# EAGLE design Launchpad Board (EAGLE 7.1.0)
CNAME: Bristol Community College; CREVISION: v1r0; DESIGNER: J. Brian
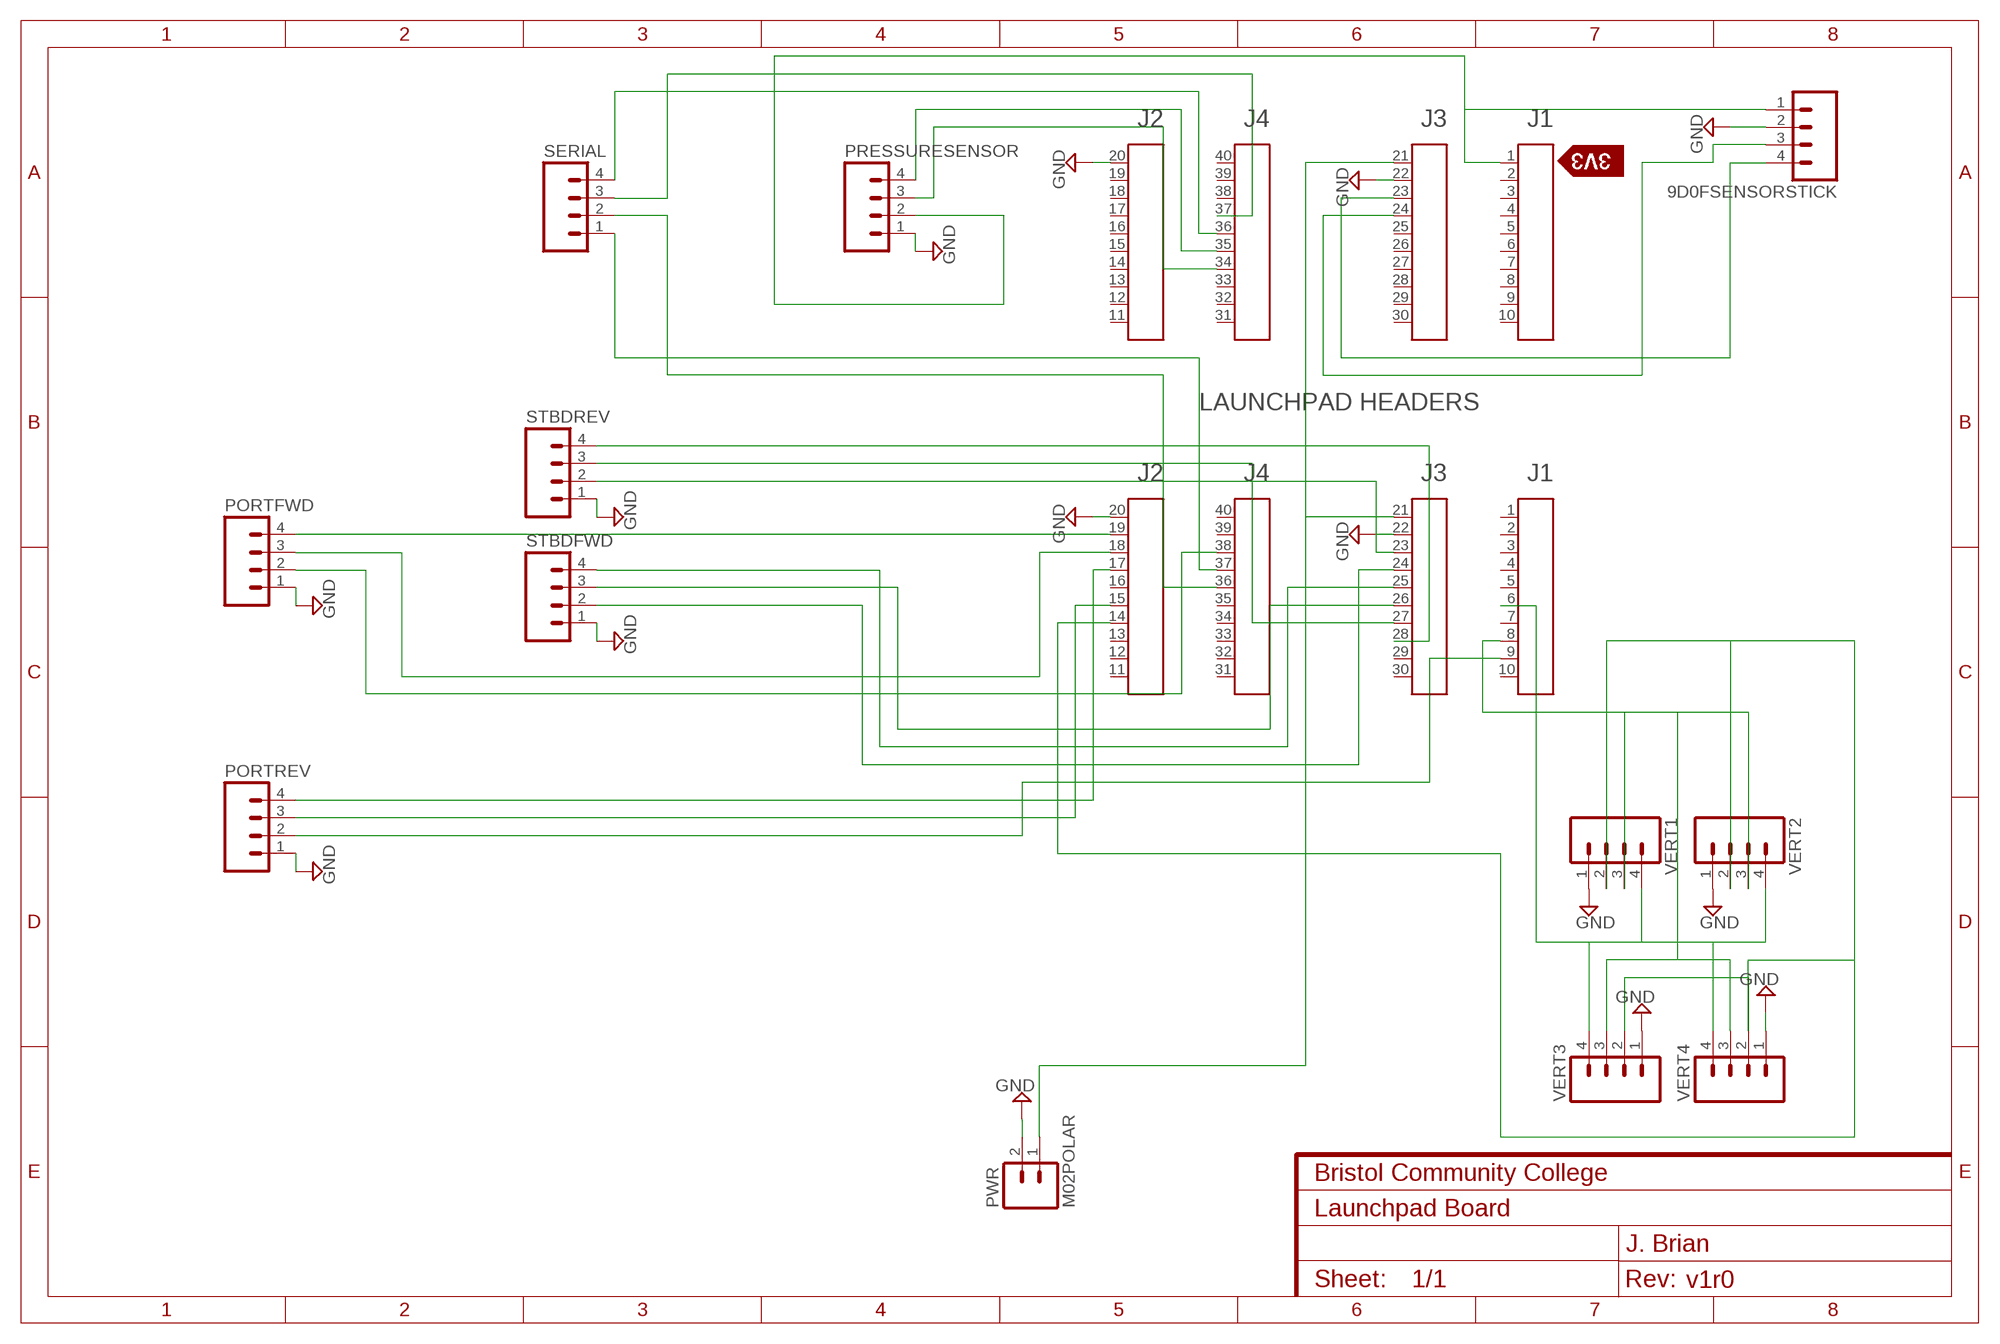
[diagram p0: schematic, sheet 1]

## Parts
9D0FSENSORSTICK  M04PTH  [1X04]
A1  HEADER4X10-BOOSTERPACK  [4X10-BOOSTERPACK]
A2  HEADER4X10-BOOSTERPACK  [4X10-BOOSTERPACK]
PORTFWD  M04POLAR_LOCK  [MOLEX-1X4_LOCK]
PORTREV  M04POLAR_LOCK  [MOLEX-1X4_LOCK]
PRESSURESENSOR  M04POLAR  [MOLEX-1X4]
PWR  M02POLAR  [MOLEX-1X2]
SERIAL  M04POLAR_LOCK  [MOLEX-1X4_LOCK]
STBDFWD  M04POLAR_LOCK  [MOLEX-1X4_LOCK]
STBDREV  M04POLAR_LOCK  [MOLEX-1X4_LOCK]
U$3  SILK_3V3_TAG  [SILK_3V3_TAG]
VERT1  M04POLAR_LOCK  [MOLEX-1X4_LOCK]
VERT2  M04POLAR_LOCK  [MOLEX-1X4_LOCK]
VERT3  M04POLAR_LOCK  [MOLEX-1X4_LOCK]
VERT4  M04POLAR_LOCK  [MOLEX-1X4_LOCK]

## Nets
GND: 9D0FSENSORSTICK.2 A1.20 A1.22 A2.20 A2.22 PORTFWD.1 PORTREV.1 PRESSURESENSOR.1 PWR.2 STBDFWD.1 STBDREV.1 VERT1.1 VERT2.1 VERT3.1 VERT4.1
N$1: A1.21 A2.21 PWR.1
N$2: 9D0FSENSORSTICK.1 A1.1 PRESSURESENSOR.2
N$3: 9D0FSENSORSTICK.3 A1.24
N$5: A2.38 PORTFWD.2
N$6: A2.9 PORTREV.2
N$7: A1.35 PRESSURESENSOR.4
N$8: A2.14 VERT1.2 VERT2.2 VERT3.2 VERT4.2
N$9: A2.8 VERT1.3 VERT2.3 VERT3.3 VERT4.3
N$10: A2.24 STBDFWD.2
N$11: A2.23 STBDREV.2
N$12: A2.25 STBDFWD.4
N$13: A2.6 VERT1.4 VERT2.4 VERT3.4 VERT4.4
N$14: A2.18 PORTFWD.3
N$15: A2.26 STBDFWD.3
N$16: A2.27 STBDREV.3
N$17: A2.28 STBDREV.4
N$18: A2.15 PORTREV.3
N$19: A1.34 PRESSURESENSOR.3
N$20: A2.17 PORTREV.4
N$21: A2.19 PORTFWD.4
N$23: A2.36 SERIAL.2
N$24: A1.36 SERIAL.4
N$25: A1.37 SERIAL.3
N$27: 9D0FSENSORSTICK.4 A1.23
N$32: A2.37 SERIAL.1
Unconnected: A1.2 A1.3 A1.4 A1.5 A1.6 A1.7 A1.8 A1.9 A1.10 A1.11 A1.12 A1.13 A1.14 A1.15 A1.16 A1.17 A1.18 A1.19 A1.25 A1.26 A1.27 A1.28 A1.29 A1.30 A1.31 A1.32 A1.33 A1.38 A1.39 A1.40 A2.1 A2.2 A2.3 A2.4 A2.5 A2.7 A2.10 A2.11 A2.12 A2.13 A2.16 A2.29 A2.30 A2.31 A2.32 A2.33 A2.34 A2.35 A2.39 A2.40

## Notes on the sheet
- LAUNCHPAD HEADERS

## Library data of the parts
9D0FSENSORSTICK PORTFWD PORTREV PRESSURESENSOR SERIAL STBDFWD STBDREV VERT1-VERT4 = SparkFun-Connectors:M04: Header 4 Standard 4-pin 0.1" header. Use with straight break away headers (SKU : PRT-00116), right angle break away headers (PRT-00553), swiss pins (PRT-00743), machine pins (PRT-00117), and female headers (PRT-00115). Molex polarized connector foot print use with SKU : PRT-08231 with associated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
A1 A2 = EAGLE_BoosterPack_Library:HEADER4X10-BOOSTERPACK
PWR = SparkFun-Connectors:M02: Standard 2-pin 0.1" header. Use with
U$3 = Public_BP_Library:SILK_3V3_TAG

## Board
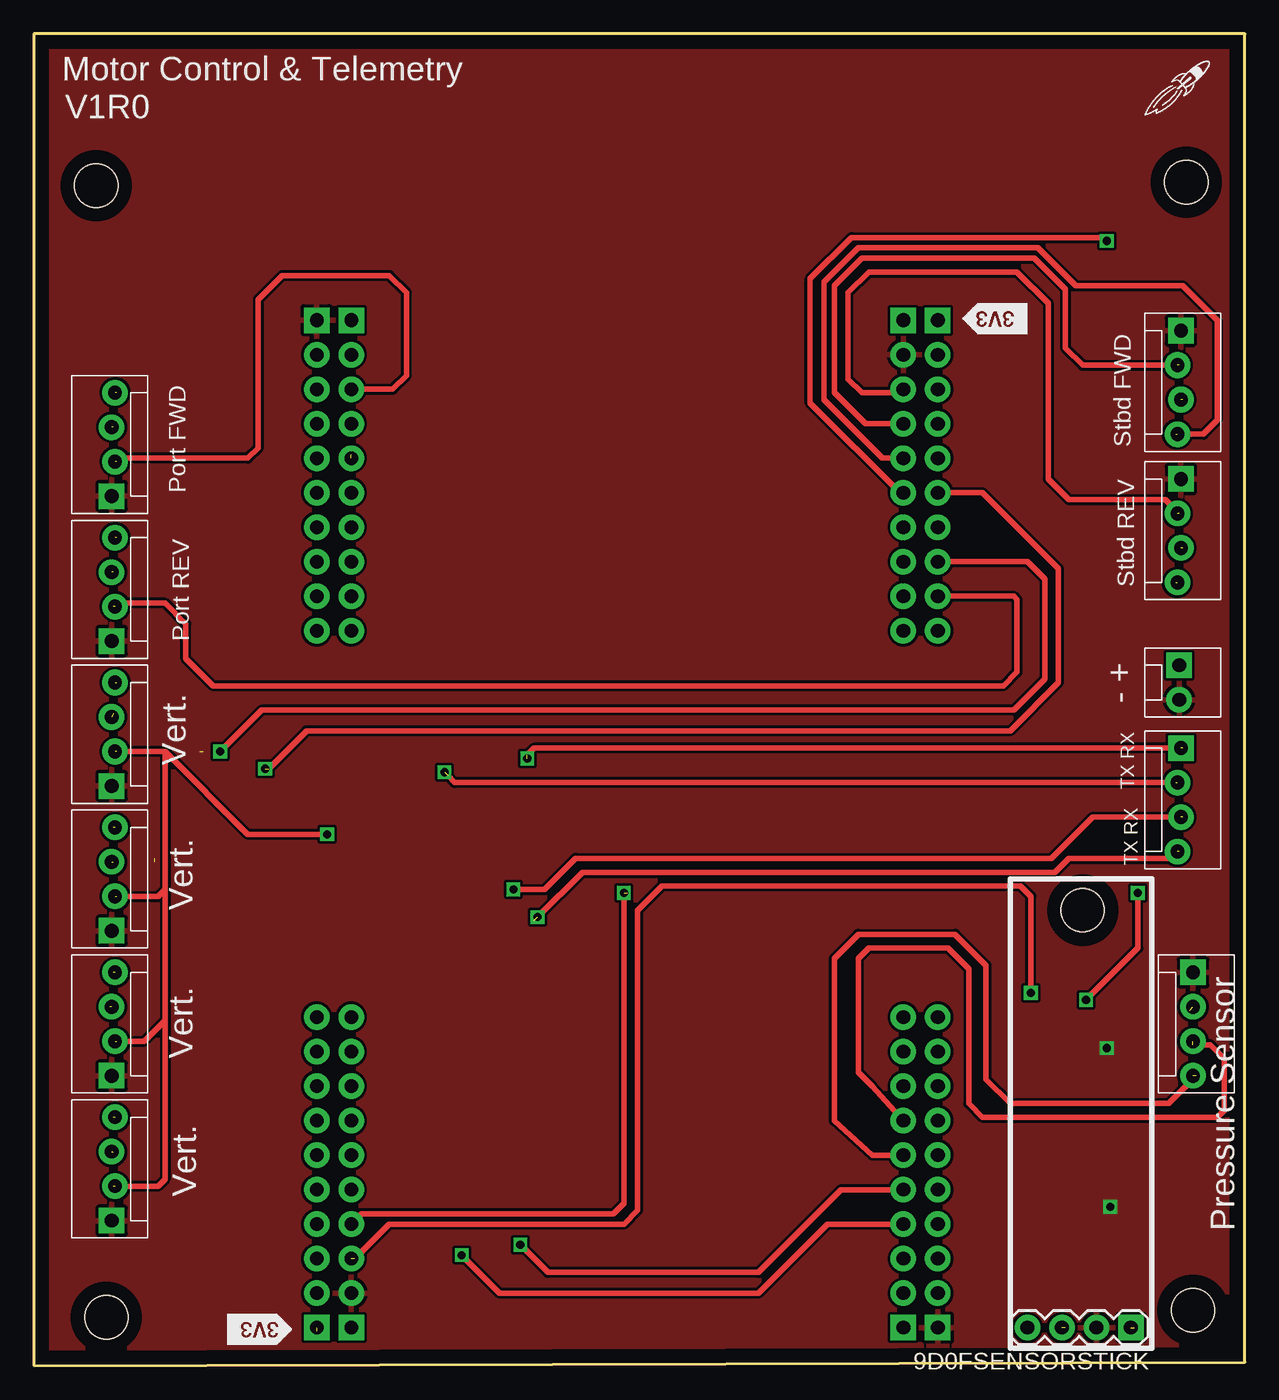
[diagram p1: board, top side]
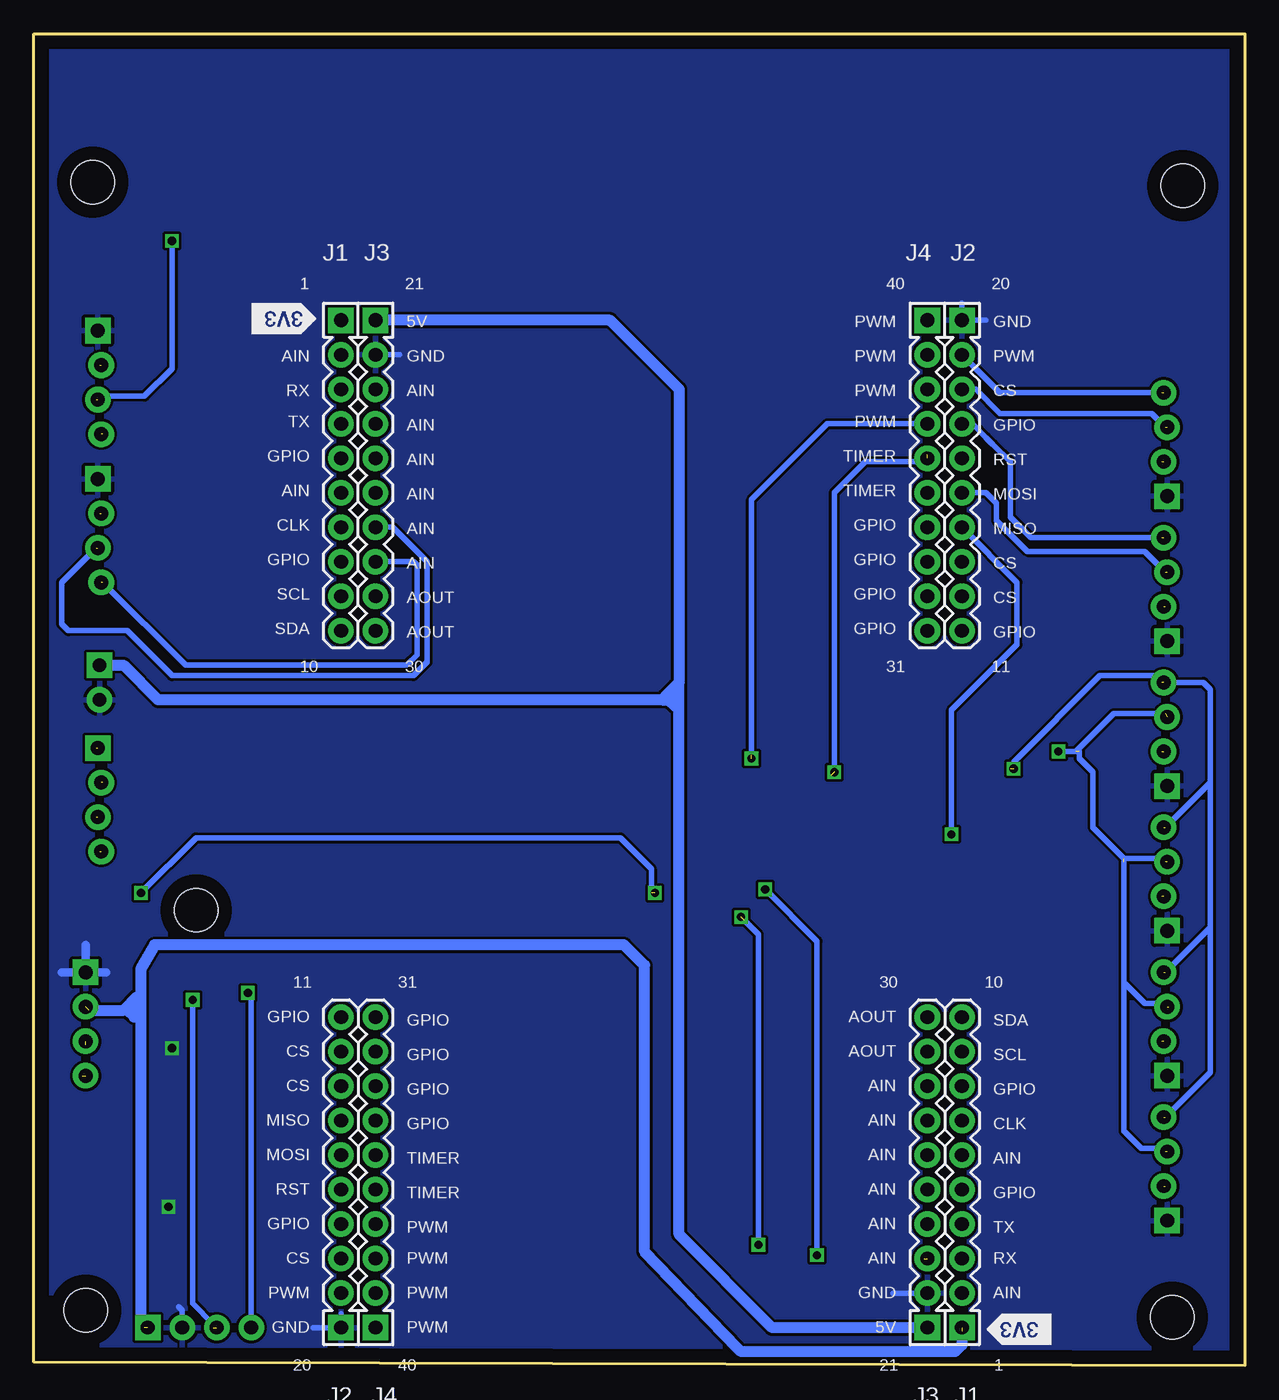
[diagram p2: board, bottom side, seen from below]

Size 89.15 x 98.04 mm. Coordinates in mm from the lower left corner, seen from the top.
Outline: 0,0 89.15,0.25 89.15,98.04 0,98.04 0,0
Copper layers (1*16): Top 0.035mm / dielectric 1.5mm / Bottom 0.035mm
Design rules "default": minimum track width 10mil, minimum drill 24mil, track to track 8mil, track to pad 8mil, pad to pad 8mil, via to via 8mil, smd to smd 8mil, copper to edge 40mil, drill to drill 8mil, minimum pad ring 10mil, minimum via ring 8mil, stop-mask expansion 4mil, vias tented up to drill 0mil, thermal gap 10mil
Holes 3.2 mm at 4.57,86.87 84.84,87.12 85.34,4.06 5.33,3.56 77.22,33.53

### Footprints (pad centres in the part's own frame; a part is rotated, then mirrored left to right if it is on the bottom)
1X04 = drill 1.016 pad 1.88 square: 1 0,0 | drill 1.016 pad 1.88: 2 2.54,0; 3 5.08,0; 4 7.62,0
4X10-BOOSTERPACK = drill 1.016 pad 1.88 square: 1 0,10.16; 20 45.72,10.16; 21 2.54,10.16; 40 43.18,10.16 | drill 1.016 pad 1.88: 2 0,7.62; 3 0,5.08; 4 0,2.54; 5 0,0; 6 0,-2.54; 7 0,-5.08; 8 0,-7.62; 9 0,-10.16; 10 0,-12.7; 11 45.72,-12.7; 12 45.72,-10.16; 13 45.72,-7.62; 14 45.72,-5.08; 15 45.72,-2.54; 16 45.72,0; 17 45.72,2.54; 18 45.72,5.08; 19 45.72,7.62; 22 2.54,7.62; 23 2.54,5.08; 24 2.54,2.54; 25 2.54,0; 26 2.54,-2.54; 27 2.54,-5.08; 28 2.54,-7.62; 29 2.54,-10.16; 30 2.54,-12.7; 31 43.18,-12.7; 32 43.18,-10.16; 33 43.18,-7.62; 34 43.18,-5.08; 35 43.18,-2.54; 36 43.18,0; 37 43.18,2.54; 38 43.18,5.08; 39 43.18,7.62
MOLEX-1X4_LOCK = drill 1.016 pad 1.88 square: 1 0,0.127 | drill 1.016 pad 1.88: 2 2.54,-0.127; 3 5.08,0.127; 4 7.62,-0.127
MOLEX-1X4 = drill 1.016 pad 1.88 square: 1 0,0 | drill 1.016 pad 1.88: 2 2.54,0; 3 5.08,0; 4 7.62,0
MOLEX-1X2 = drill 1.016 pad 1.88 square: 1 0,0 | drill 1.016 pad 1.88: 2 2.54,0

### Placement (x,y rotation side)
9D0FSENSORSTICK  80.77,2.79 180 top
A1  20.83,12.95 180 bottom
A2  66.55,66.8 0 bottom
PORTFWD  5.84,64.01 90 top
PORTREV  5.84,53.34 90 top
PRESSURESENSOR  85.34,28.96 270 top
PWR  84.33,51.56 270 top
SERIAL  84.33,45.47 270 top
STBDFWD  84.33,76.2 270 top
STBDREV  84.33,65.28 270 top
U$1  SILK_3V3_TAG  [SILK_3V3_TAG]  73.15,78.23 180 top
U$2  [LOGO-ROCKET]  84.33,94.23 0 top
U$3  14.22,3.81 180 bottom
VERT1  5.84,42.67 90 top
VERT2  5.84,10.67 90 top
VERT3  5.84,32 90 top
VERT4  5.84,21.34 90 top

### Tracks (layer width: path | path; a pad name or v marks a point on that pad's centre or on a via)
GND  (via drill 0.6)
  Bottom 0.406: 20.83,78.23 A2.20 19.05,76.96 | A2.22 62.23,74.42 | A1.22 25.91,5.33 | 66.55,3.81 A1.20 68.58,2.79 | 9D0FSENSORSTICK.2 78.23,4.06 78.49,4.32
  Bottom 0.61: PRESSURESENSOR.1 85.34,30.99 | PRESSURESENSOR.1 87.12,28.96 | PRESSURESENSOR.1 83.82,28.96
  other vias: 79.25,11.68 78.99,23.37
  pour Top: 10.67,98.3 89.41,97.79 89.41,0.25 73.91,0.51 0,0 0,97.79
  pour Bottom: 10.67,98.3 89.41,98.04 89.41,0.25 -0.25,0.25 0.25,98.04
N$1
  Bottom 0.813: A1.21 34.8,2.79 41.66,9.65 41.66,50.29 | 63.75,76.96 46.74,76.96 41.66,71.88 41.66,50.29 | 63.75,76.96 64.01,77.22 | A2.21 63.75,76.96 | 42.93,49.02 42.42,49.02 41.91,48.51 | 41.66,50.29 42.93,49.02 | PWR.1 82.55,51.56 80.01,49.02 42.93,49.02
N$2  (3 unrouted)
  Bottom 0.813: 20.83,2.54 20.83,1.52 21.34,1.02 37.08,1.02 37.34,1.27 44.2,8.38 44.2,29.46 45.72,30.99 80.26,30.99 81.28,29.21 81.28,25.65 | 85.09,26.16 82.55,26.16 81.53,27.18 81.53,25.91 81.28,25.65 | 81.28,25.65 81.28,3.05 81.03,2.79 | 81.28,25.65 81.79,25.65 82.3,26.16
N$3  (via drill 0.6)  (2 unrouted)
  Top 0.406: v43.43,34.8 43.43,11.94 42.67,11.18 24.13,11.18 A1.24 | v81.28,34.8 81.28,30.73 77.72,27.18 77.47,27.18 v77.47,26.92
  Bottom 0.406: v81.28,34.8 77.22,38.86 45.97,38.86 43.69,36.58 43.69,34.8 43.43,34.54 | 75.95,2.79 75.95,3.05 77.47,4.57 v77.47,26.92 77.47,27.18
N$4
  Bottom 0.813: 42.67,49.28 41.91,50.04
N$5  (1 unrouted)
  Top 0.406: A2.38 26.42,71.88 27.43,72.9 27.43,78.99 26.16,80.26 18.29,80.26 16.51,78.49 16.51,67.56 15.75,66.8 6.35,66.8 6.1,66.55
N$6  (1 unrouted)
  Top 0.406: A2.9 72.14,56.64 72.39,56.39 72.39,51.05 71.37,50.04 13.21,50.04 11.18,52.07 11.18,54.61 9.65,56.13 6.1,56.13 5.84,55.88
N$7  (1 unrouted)
  Top 0.406: A1.35 61.72,15.49 58.93,18.03 58.93,29.97 60.71,31.75 67.82,31.75 70.1,29.46 70.1,21.08 71.88,19.3 83.57,19.3 85.6,21.34
N$8  (via drill 0.6)  (4 unrouted)
  Top 0.406: v21.59,39.12 15.75,39.12 9.65,45.21 | 9.65,45.21 6.1,45.21 | 9.65,45.21 9.65,35.05 | 9.65,35.05 9.65,25.4 | 9.65,25.4 9.65,13.72 9.14,13.21 5.84,13.21 | 6.1,34.54 9.14,34.54 9.65,35.05 | 6.1,23.88 8.13,23.88 9.65,25.4
  Bottom 0.406: v21.59,39.12 21.59,48.26 16.76,53.09 16.76,57.66 A2.14
N$9  (via drill 0.6)  (6 unrouted)
  Top 0.406: A2.8 73.15,59.18 74.42,57.91 74.42,50.55 72.14,48.26 16.76,48.26 v13.72,45.21
  Bottom 0.406: 8.89,37.08 8.89,28.19 | 8.89,28.19 7.37,26.67 5.84,26.67 5.59,26.42 | 8.89,28.19 8.89,17.27 7.62,16 6.1,16 5.84,15.75 | v13.72,45.21 12.45,45.21 9.65,48.01 5.84,48.01 | 12.19,45.21 12.19,44.7 11.18,43.69 11.18,39.62 8.89,37.34 6.1,37.34 5.84,37.08
N$10  (1 unrouted)
  Top 0.406: 84.33,73.66 77.22,73.66 75.95,74.93 75.95,79.25 73.66,81.53 60.96,81.53 58.93,79.5 58.93,71.63 61.21,69.34 A2.24
N$11  (1 unrouted)
  Top 0.406: 84.33,62.74 83.31,63.75 76.2,63.75 74.68,65.28 74.68,78.23 72.39,80.52 61.47,80.52 59.94,78.99 59.94,72.64 60.96,71.63 64.01,71.63 A2.23
N$12  (1 unrouted)
  Top 0.406: A2.25 62.48,66.8 58.17,71.12 58.17,79.76 60.71,82.3 73.91,82.3 76.71,79.5 84.58,79.5 87.12,76.96 87.12,69.6 86.11,68.58 84.07,68.58
N$13  (via drill 0.6)  (5 unrouted)
  Top 0.406: A2.6 69.85,64.26 75.44,58.67 75.44,50.29 71.88,46.74 20.07,46.74 17.27,43.94
  Bottom 0.406: v17.02,43.94 17.02,44.45 10.67,50.8 6.6,50.8 6.1,50.29 3.05,50.29 2.54,49.78 2.54,42.93 | 2.54,42.93 5.84,39.62 | 2.54,42.93 2.54,32.26 | 2.54,32.26 5.84,28.96 | 2.54,32.26 2.54,21.59 5.84,18.29
N$14  (1 unrouted)
  Bottom 0.406: A2.18 19.81,71.88 18.03,70.1 6.86,70.1 5.84,69.09
N$15  (via drill 0.6)  (1 unrouted)
  Top 0.406: A2.26 63.75,64.26 57.15,70.87 57.15,80.01 60.2,83.06 78.74,83.06 v78.99,82.8
  Bottom 0.406: v78.99,82.8 78.99,73.41 81.03,71.37 84.33,71.37 84.58,71.12
N$16  (1 unrouted)
  Bottom 0.406: A2.27 62.74,61.72 60.2,59.18 60.2,51.82 61.21,50.8 78.99,50.8 82.3,54.1 86.61,54.1 87.12,54.61 87.12,57.66 84.58,60.2
N$17  (1 unrouted)
  Bottom 0.406: A2.28 61.21,59.18 60.96,58.93 60.96,52.32 61.72,51.56 77.98,51.56 84.07,57.66
N$18  (1 unrouted)
  Bottom 0.406: A2.15 19.05,64.26 18.29,63.5 18.29,62.23 16,59.94 7.37,59.94 5.84,58.42
N$19  (1 unrouted)
  Top 0.406: A1.34 61.72,20.57 60.71,21.59 60.71,29.97 61.47,30.73 67.31,30.73 68.83,29.21 68.83,19.3 69.85,18.29 87.12,18.29 87.63,18.8 87.63,22.61 86.61,23.62 85.34,23.62 85.09,23.88
N$20  (1 unrouted)
  Bottom 0.406: 6.1,60.96 15.75,60.96 17.27,62.48 17.27,66.55 18.54,67.82 19.05,68.33 20.07,69.34 A2.17
N$21  (1 unrouted)
  Bottom 0.406: 6.1,71.63 18.03,71.63 A2.19
N$23  (via drill 0.6)  (3 unrouted)
  Top 0.406: 84.07,42.93 30.99,42.93 30.48,43.43
  Bottom 0.406: v30.23,43.69 30.23,64.26 27.94,66.55 23.88,66.55 23.37,67.06
N$24  (via drill 0.6)  (2 unrouted)
  Top 0.406: A1.36 59.44,12.95 53.34,6.86 37.85,6.86 v35.81,8.89 | v37.08,33.02 40.39,36.32 75.18,36.32 76.2,37.34 83.82,37.34 84.33,37.85
  Bottom 0.406: v35.81,8.89 35.81,31.75 36.83,32.77
N$25  (via drill 0.6)  (1 unrouted)
  Top 0.406: A1.37 58.42,10.41 53.34,5.33 34.29,5.33 v31.5,8.13 | v35.31,35.05 37.59,35.05 39.88,37.34 74.93,37.34 77.98,40.39 84.58,40.39
  Bottom 0.406: v31.5,8.13 31.5,31.24 v35.31,35.05
N$27  (via drill 0.6)  (1 unrouted)
  Top 0.406: 73.41,3.3 73.15,3.05 | 73.15,3.05 72.9,2.79 | 73.15,3.05 9D0FSENSORSTICK.4 | v73.41,27.43 73.41,34.54 72.64,35.31 46.23,35.31 44.45,33.53 44.45,11.43 43.43,10.41 26.16,10.41 23.62,7.87
  Bottom 0.406: 9D0FSENSORSTICK.4 73.15,27.18 v73.41,27.43
N$32  (via drill 0.6)  (2 unrouted)
  Top 0.406: 84.58,45.47 36.83,45.47 36.32,44.96
  Bottom 0.406: v36.32,44.7 36.32,63.75 30.73,69.34 A2.37

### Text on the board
tPlace: Motor Control & Telemetry | V1R0
tNames: Stbd FWD | Stbd REV | Port FWD | Port REV | - + | Vert. | TX RX | TX RX | Vert. | Vert. | Vert. | Pressure Sensor

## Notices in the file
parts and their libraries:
SparkFun-Connectors: Licensing: Creative Commons ShareAlike 4.0 International - https://creativecommons.org/licenses/by-sa/4.0
